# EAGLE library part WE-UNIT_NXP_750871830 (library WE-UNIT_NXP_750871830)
Off-Line Transformer WE-Unit NXP - Nominal input voltage: 85-265 VAC - Operating temperature: -40°C to +125 °C - Isolation voltage 4 kVAC -- Especially designed for several ICs from NXP TEA1523P -- Universal input -- Smart meters -- Dimmable 12 V LED driver -- Offline-switch mode power supplies
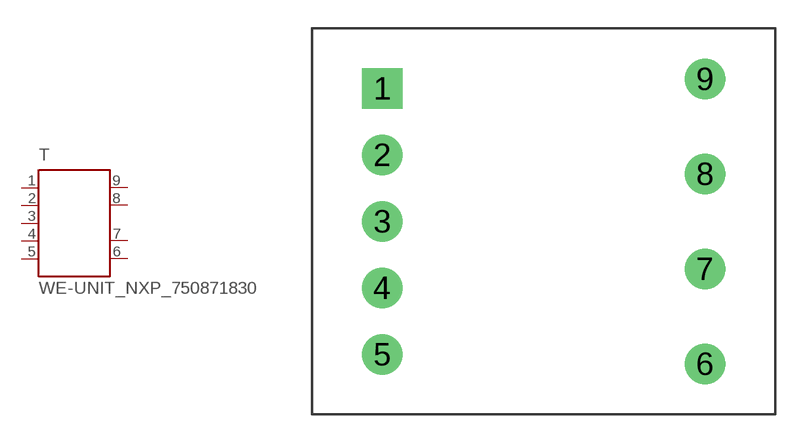
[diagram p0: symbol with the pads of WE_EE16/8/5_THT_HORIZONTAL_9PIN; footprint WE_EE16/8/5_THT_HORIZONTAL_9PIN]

Designator prefix T

## WE-UNIT_NXP_750871830 (MPN: 750871830; OC_FARNELL: 1849055; OC_NEWARK: 13T9847; PACKAGE: EE16_8_5_NXP; SUPPLIER: Würth Elektronik eiSos GmbH)  [WE_EE16/8/5_THT_HORIZONTAL_9PIN]
1  5  pas
2  4  pas
3  3  pas
4  2  pas
5  1  pas
6  9  pas
7  8  pas
8  7  pas
9  6  pas

## Footprint WE_EE16/8/5_THT_HORIZONTAL_9PIN (pad centres in mm)
Transformer, EE16/8/5 THT Horizontal 9 Pin
drill 1.42 square: 1 -8.5,7
drill 1.42: 2 -8.5,3.5; 3 -8.5,0; 4 -8.5,-3.5; 5 -8.5,-7; 6 8.5,-7.5; 7 8.5,-2.5; 8 8.5,2.5; 9 8.5,7.5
